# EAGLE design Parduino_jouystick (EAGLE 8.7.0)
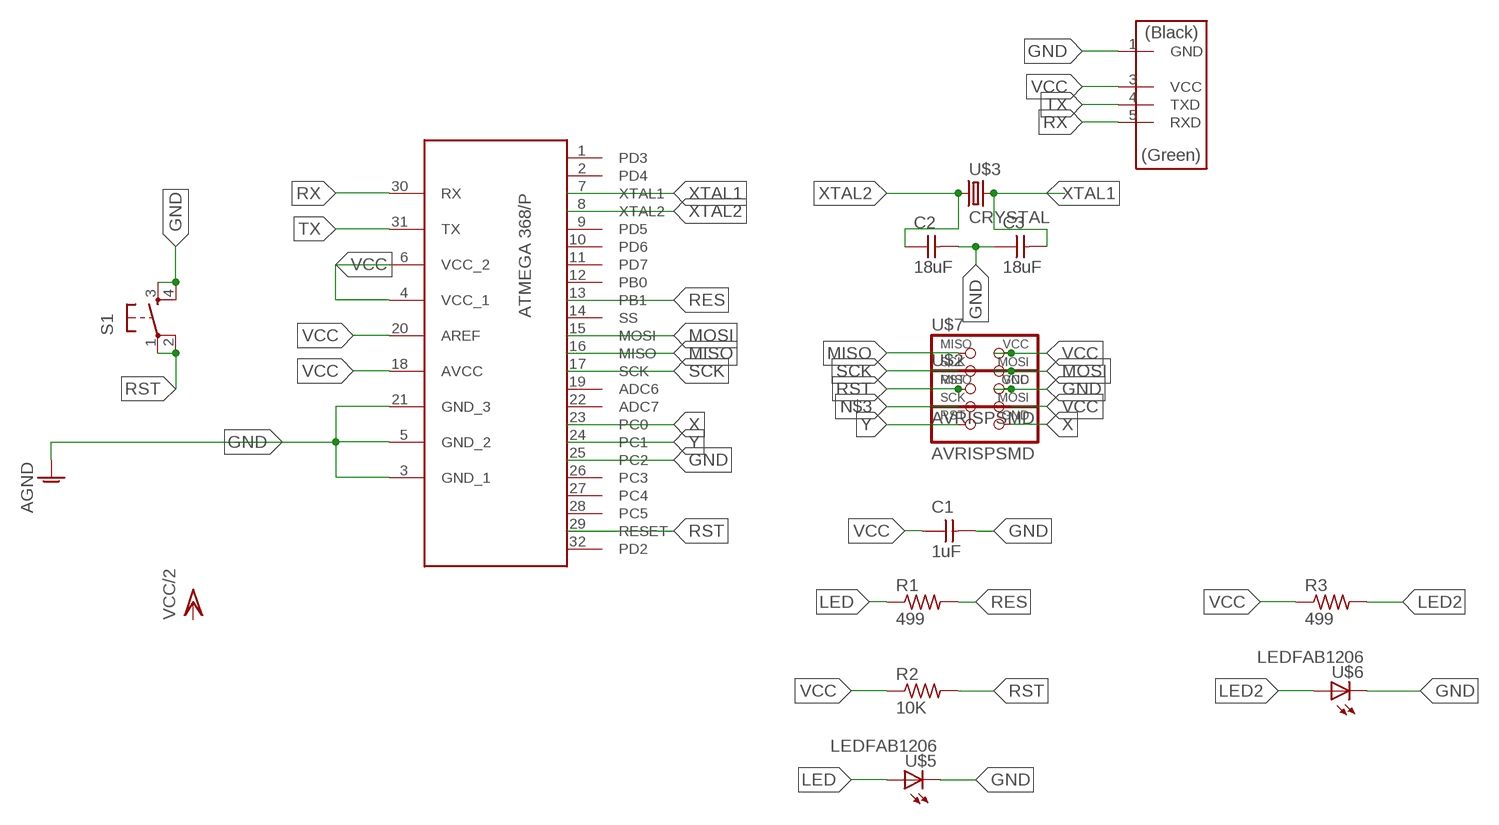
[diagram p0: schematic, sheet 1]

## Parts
C1  1uF  CAP-UNPOLARIZEDFAB  [C1206FAB]
C2  18uF  CAP-UNPOLARIZEDFAB  [C1206FAB]
C3  18uF  CAP-UNPOLARIZEDFAB  [C1206FAB]
R1  499  RES-US1206FAB  [R1206FAB]
R2  10K  RES-US1206FAB  [R1206FAB]
R3  499  RES-US1206FAB  [R1206FAB]
S1  6MM_SWITCH6MM_SWITCH  [6MM_SWITCH]
U$1  ATMEGA368  [ATMEGA328/P]
U$2  AVRISPSMD  [2X03SMD]
U$3  CRYSTAL  [2-SMD-5X3MM]
U$4  FTDI_2  [1X06SMD_2]
U$5  LEDFAB1206  [LED1206FAB]
U$6  LEDFAB1206  [LED1206FAB]
U$7  AVRISPSMD  [2X03SMD]

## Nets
GND: C1.2 C2.2 C3.1 S1.3(S) S1.4(S1) U$1.3(GND_1) U$1.5(GND_2) U$1.21(GND_3) U$1.25(PC2) U$2.2(VCC) U$4.1(GND) U$5.2(C) U$6.2(C) U$7.6(GND) ; supply symbol labelled AGND
LED: R1.1 U$5.1(A)
LED2: R3.2 U$6.1(A)
MISO: U$1.16(MISO) U$7.1(MISO)
MOSI: U$1.15(MOSI) U$7.4(MOSI)
N$3: U$2.3(SCK)
RES: R1.2 U$1.13(PB1)
RST: R2.2 S1.1(P) S1.2(P1) U$1.29(RESET) U$2.1(MISO) U$7.5(RST)
RX: U$1.30(RX) U$4.5(RXD)
SCK: U$1.17(SCK) U$7.3(SCK)
TX: U$1.31(TX) U$4.4(TXD)
VCC: C1.1 R2.1 R3.1 U$1.4(VCC_1) U$1.6(VCC_2) U$1.18(AVCC) U$1.20(AREF) U$2.4(MOSI) U$4.3(VCC) U$7.2(VCC)
X: U$1.23(PC0) U$2.6(GND)
XTAL1: C3.2 U$1.7(XTAL1) U$3.P$2
XTAL2: C2.1 U$1.8(XTAL2) U$3.P$1
Y: U$1.24(PC1) U$2.5(RST)
Unconnected: U$1.1(PD3) U$1.2(PD4) U$1.9(PD5) U$1.10(PD6) U$1.11(PD7) U$1.12(PB0) U$1.14(SS) U$1.19(ADC6) U$1.22(ADC7) U$1.26(PC3) U$1.27(PC4) U$1.28(PC5) U$1.32(PD2)

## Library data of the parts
C1-C3 = fab:CAP-UNPOLARIZED
R1-R3 = fab:RES-US: Resistor (US Symbol)
S1 = fab:6MM_SWITCH: OMRON SWITCH
U$1 = Paul:ATMEGA368
U$2 U$7 = 01fab:AVRISP
U$3 = 01fab:CRYSTAL
U$4 = fab:FTDI_2
U$5 U$6 = fab:LED: LED

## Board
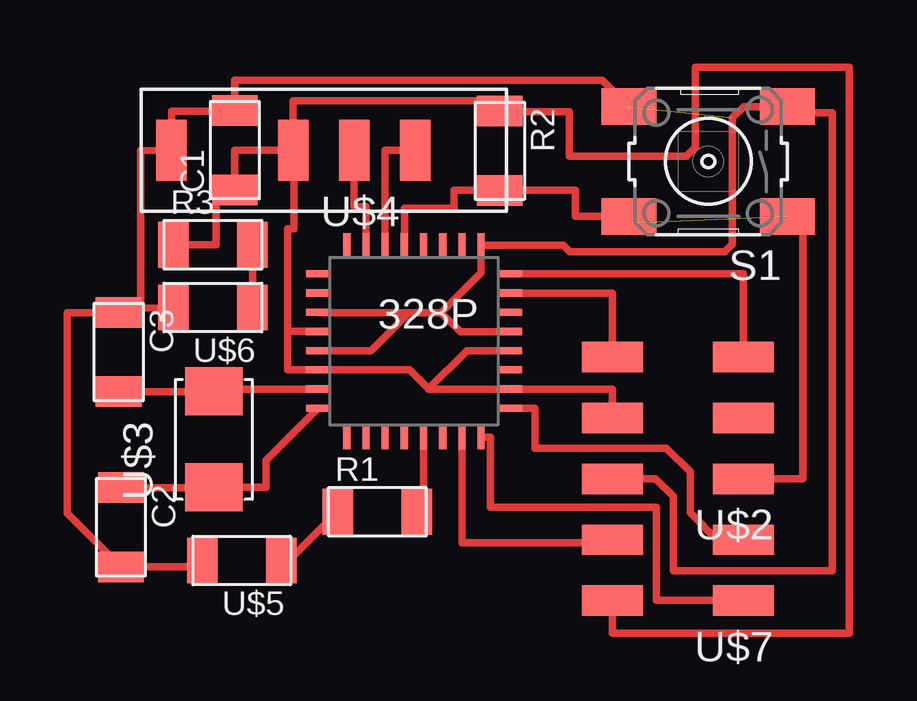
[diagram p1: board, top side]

No outline drawn. Coordinates in mm, seen from the top.
Copper layers (1*16): Top 0.035mm / dielectric 1.5mm / Bottom 0.035mm
Design rules "default *": minimum track width 6mil, minimum drill 0.35mm, track to track 16mil, track to pad 16mil, pad to pad 16mil, via to via 16mil, smd to smd 16mil, copper to edge 40mil, drill to drill 6mil, minimum pad ring 10mil, minimum via ring 8mil, stop-mask expansion 4mil, vias tented up to drill 0mil, thermal gap 10mil

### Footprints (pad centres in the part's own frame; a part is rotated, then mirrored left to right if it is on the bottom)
C1206FAB = smd 1.27 x 1.905: 1 -1.651,0; 2 1.651,0
R1206FAB = smd 1.27 x 1.905: 1 -1.651,0; 2 1.651,0
6MM_SWITCH = smd 2.286 x 1.524: 1 -3.302,2.286; 2 3.302,2.286; 3 -3.302,-2.286; 4 3.302,-2.286
ATMEGA328/P = smd 1 x 0.3: 1 -4,2.8; 2 -4,2; 3 -4,1.2; 4 -4,0.4; 5 -4,-0.4; 6 -4,-1.2; 7 -4,-2; 8 -4,-2.8; 17 4,-2.8; 18 4,-2; 19 4,-1.2; 20 4,-0.4; 21 4,0.4; 22 4,1.2; 23 4,2; 24 4,2.8 | smd 0.3 x 1: 9 -2.8,-4; 10 -2,-4; 11 -1.2,-4; 12 -0.4,-4; 13 0.4,-4; 14 1.2,-4; 15 2,-4; 16 2.8,-4; 25 2.8,4; 26 2,4; 27 1.2,4; 28 0.4,4; 29 -0.4,4; 30 -1.2,4; 31 -2,4; 32 -2.8,4
2X03SMD = smd 2.54 x 1.27: 1 -2.54,2.54; 2 2.92,2.54; 3 -2.54,0; 4 2.92,0; 5 -2.54,-2.54; 6 2.92,-2.54
2-SMD-5X3MM = smd 2 x 2.4: P$1 -2,0; P$2 2,0
1X06SMD_2 = smd 2.54 x 1.27: 1 0,6.35; 3 0,1.27; 4 0,-1.27; 5 0,-3.81
LED1206FAB = smd 1.27 x 1.905: 1 -1.651,0; 2 1.651,0

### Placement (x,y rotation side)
C1  7.38,19.13 90 top
C2  2.63,3.42 270 top
C3  2.54,10.72 270 top
R1  13.32,4.06 0 top
R2  18.43,19.1 270 top
R3  6.46,15.19 0 top
S1  27.11,18.66 180 top
U$1  14.85,11.18 0 top
U$2  26.04,7.98 180 top
U$3  6.5,7.07 90 top
U$4  11.09,19.13 90 top
U$5  7.67,2.03 180 top
U$6  6.46,12.57 180 top
U$7  26.04,2.9 180 top

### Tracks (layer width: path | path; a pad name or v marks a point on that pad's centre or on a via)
GND  (1 unrouted)
  Top 0.305: U$6.2 3.61,12.55 | 3.61,12.55 3.45,12.55 3.45,19.1 U$4.1 4.74,20.75 7.38,20.75 C1.2 7.38,21.6 7.38,22.05 22.71,22.05 S1.4 | 3.61,12.55 2.72,12.55 C3.1 2.53,12.36 0.39,12.36 0.39,4 C2.2 5.75,1.76 U$5.2 | U$1.5 13.06,10.78 14.64,12.36 | 14.64,12.36 10.87,12.36 U$1.3 | 14.64,12.36 15.98,12.36 | 15.98,12.36 16.78,11.56 18.83,11.56 U$1.21 | U$7.6 24.92,5.44 25.66,4.7 25.66,1.61 32.28,1.61 32.28,20.69 30.67,20.69 S1.3 28.6,20.94 28.13,20.47 28.13,15.21 27.81,14.9 21.35,14.9 21.07,15.18 U$1.25 17.65,14.03 15.98,12.36
LED
  Top 0.305: U$5.1 9.64,2.03 R1.1
LED2
  Top 0.305: R3.2 U$6.1
MISO
  Top 0.305: U$1.16 18.03,7.18 18.03,4.24 24.94,4.24 24.94,0.38 28.57,0.38 U$7.1
MOSI
  Top 0.305: U$1.15 16.85,2.77 23.11,2.77 | 24.09,2.77 23.11,2.77 | 23.11,2.77 U$7.4
RES
  Top 0.305: R1.2 15.25,4.34 U$1.13
RST  (1 unrouted)
  Top 0.305: 18.43,17.14 R2.2 | R2.2 16.52,17.45 16.52,16.7 14.45,16.7 U$1.29 | R2.2 21.58,17.45 21.58,16.37 S1.2 23.98,16.1 | U$7.5 31.06,5.44 31.06,16.37 | 31.06,16.4 31.06,16.37 | 31.06,16.37 S1.1
RX
  Top 0.305: U$1.30 13.65,19.13 U$4.5
SCK
  Top 0.305: U$1.17 19.9,8.38 19.9,6.72 25.38,6.72 26.37,5.73 26.37,4.01 27.56,2.82 27.64,2.9 U$7.3
TX
  Top 0.305: U$1.31 12.85,16.76 12.36,16.76 U$4.4
VCC
  Top 0.305: U$4.3 9.82,21.18 18.43,21.18 R2.1 21.34,20.74 21.34,18.89 26.2,18.89 26.57,19.25 26.57,22.58 32.99,22.58 32.99,-1 23.11,-1 U$7.2 | U$4.3 9.84,19.13 9.84,15.85 9.59,15.85 9.59,11.58 | U$1.4 9.59,11.58 | R3.1 6.59,15.19 6.59,17.48 C1.1 7.38,19.13 U$4.3 | 9.59,11.58 9.59,9.98 U$1.6 14.66,9.98 15.46,9.18 | U$2.4 23.11,9.18 U$1.18 15.46,9.18 | U$1.20 17.05,10.78 15.46,9.18
X
  Top 0.305: U$1.23 23.11,13.18 U$2.6
XTAL1
  Top 0.305: C3.2 U$3.P$2 6.6,9.18 U$1.7
XTAL2
  Top 0.305: C2.1 U$3.P$1 8.69,5.08 8.69,6.22 U$1.8
Y
  Top 0.305: U$1.24 28.57,13.98 U$2.5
